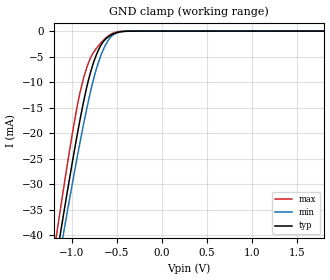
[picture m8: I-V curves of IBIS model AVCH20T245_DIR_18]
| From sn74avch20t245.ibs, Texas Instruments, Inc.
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[Model]   AVCH20T245_DIR_18
Model_type  Input
Vinl=0.5775
Vinh=1.2675
| variable   typ   min   max
C_comp   2.73pF   2.23pF   3.27pF
[Temperature Range]   40   100   -40
| Ambient temperature   25   85   -40
[Voltage range]   1.8   1.65   1.95
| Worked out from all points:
|   GND clamp passes 1 mA (typ) near -0.58 V on its own axis
[GND Clamp]
| AVCH20T245_DIR_18
|   Voltage   I(typ)   I(min)   I(max)
-4.6V     -459.2mA   -437.9mA   -484.2mA
-1.185V   -45.97mA   -49.06mA   -41.71mA
-1.155V   -42.69mA   -45.98mA   -38.17mA
-1.13V    -39.97mA   -43.42mA   -35.25mA
-1.105V   -37.28mA   -40.88mA   -32.35mA
-1.08V    -34.61mA   -38.36mA   -29.5mA
-950mV    -21.28mA   -25.63mA   -15.65mA
-840mV    -11.44mA   -15.71mA   -7.485mA
-765mV    -6.504mA   -9.869mA   -4.351mA
-695mV    -3.38mA    -5.644mA   -2.68mA
-540mV    -571.7uA   -743.1uA   -384.3uA
1.8V      129.6pA    822.2pA    26.26pA
